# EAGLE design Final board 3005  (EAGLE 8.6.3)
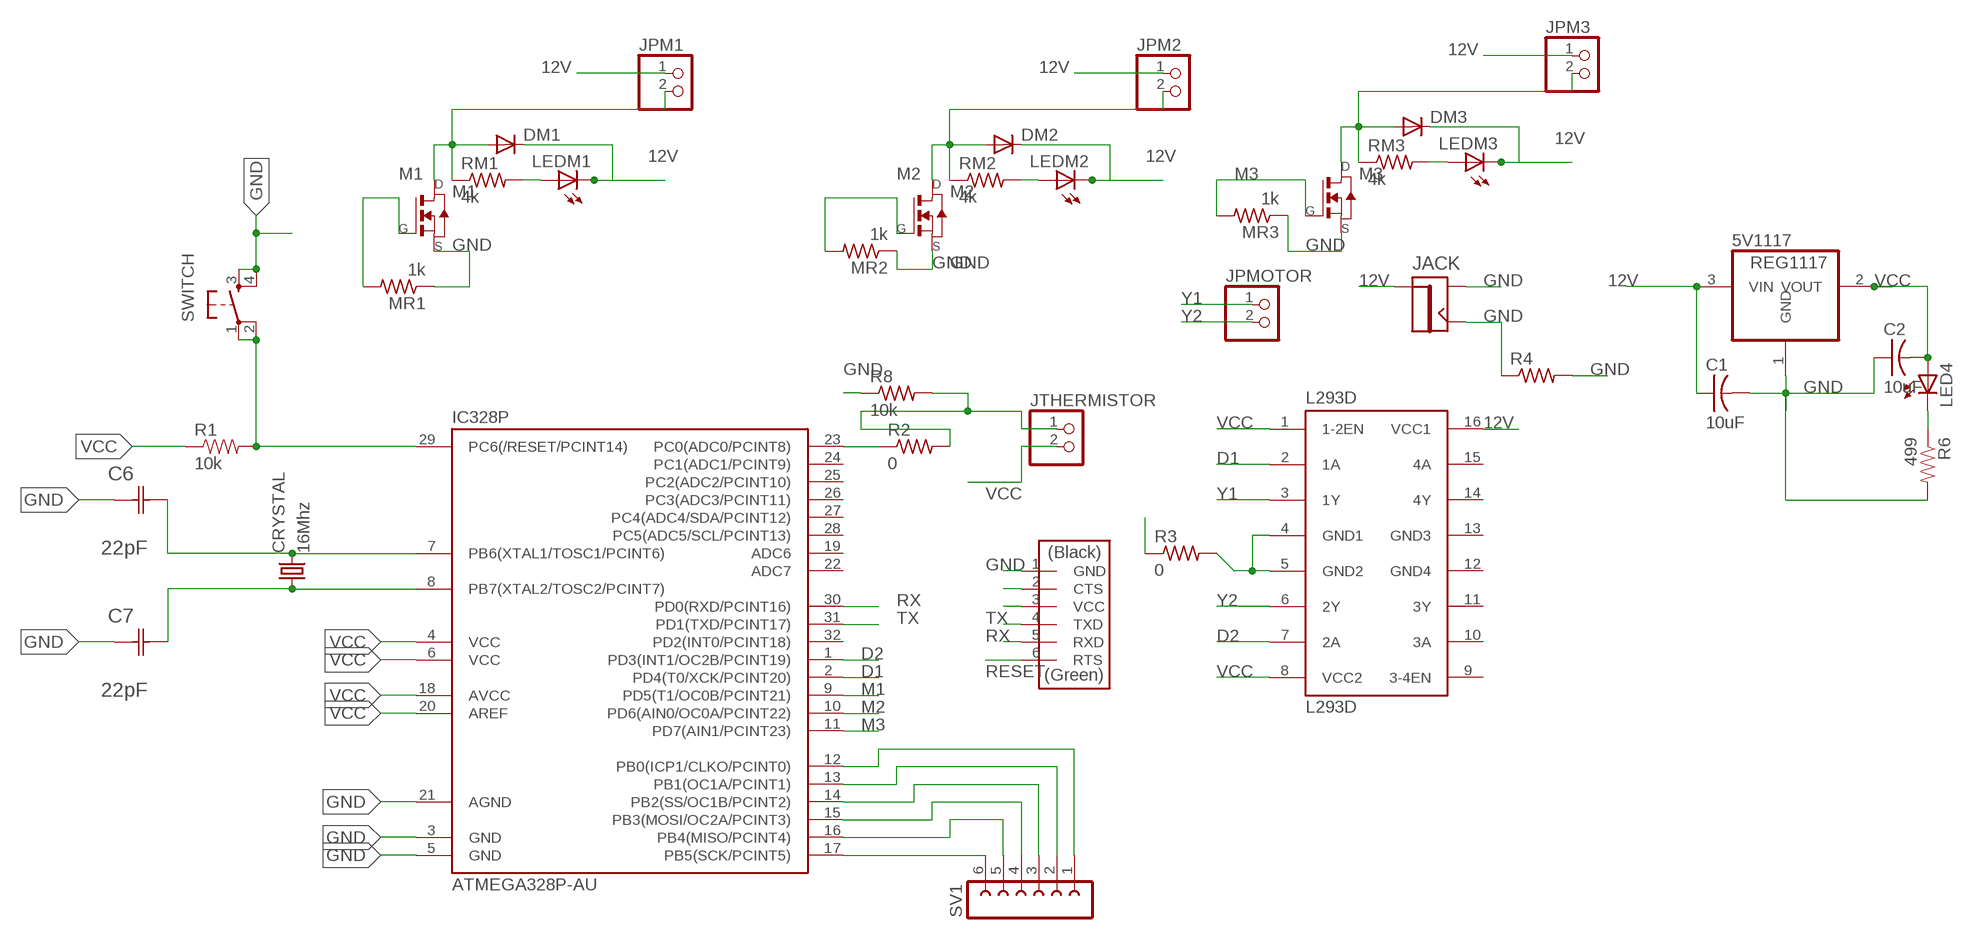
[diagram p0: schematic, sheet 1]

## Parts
5V1117  REG1117  [SOT223]
C1  10uF  CAP-US1206FAB  [C1206FAB]
C2  10uF  CAP-US1206FAB  [C1206FAB]
C6  22pF  0612ZC225MAT2A  [CAPC3216X178N]
C7  22pF  0612ZC225MAT2A  [CAPC3216X178N]
CRYSTAL  16Mhz  CSM-7X-DU  [CSM-7X-DU]
DM1  DIODESOD123  [SOD123]
DM2  DIODESOD123  [SOD123]
DM3  DIODESOD123  [SOD123]
FTDI  FTDI-SMD-HEADER  [1X06SMD]
IC328P  ATMEGA328P-AU  ATMEGA48/88/168-AU  [TQFP32-08]
JACK  JACK2.1MM  [JACK_2.1MM]
JPM1  PINHD-1X2  [1X02]
JPM2  PINHD-1X2  [1X02]
JPM3  PINHD-1X2  [1X02]
JPMOTOR  PINHD-1X2  [1X02]
JTHERMISTOR  PINHD-1X2  [1X02]
L293D  L293D  [DIL16]
LED4  LEDSMT1206  [1206]
LEDM1  LEDSMT1206  [1206]
LEDM2  LEDSMT1206  [1206]
LEDM3  LEDSMT1206  [1206]
M1  NMOSFETTO252  [TO252]
M2  NMOSFETTO252  [TO252]
M3  NMOSFETTO252  [TO252]
MR1  1k  RES-US1206FAB  [R1206FAB]
MR2  1k  RES-US1206FAB  [R1206FAB]
MR3  1k  RES-US1206FAB  [R1206FAB]
R1  10k  RESISTOR1206  [1206]
R2  0  RES-US1206FAB  [R1206FAB]
R3  0  RES-US1206FAB  [R1206FAB]
R4  RES-US1206FAB  [R1206FAB]
R6  499  RESISTOR1206  [1206]
R8  10k  RES-US1206FAB  [R1206FAB]
RM1  4k  RES-US1206  [R1206]
RM2  4k  RES-US1206  [R1206]
RM3  4k  RES-US1206  [R1206]
SV1  FE06-1  [FE06]
SWITCH  6MM_SWITCH6MM_SWITCH  [6MM_SWITCH]

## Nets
12V: 5V1117.3(VIN) C1.1 DM1.CATHODE(C) DM2.CATHODE(C) DM3.CATHODE(C) JACK.PIN JPM1.1 JPM2.1 JPM3.1 L293D.16(VCC1) LEDM1.C LEDM2.C LEDM3.C
D1: IC328P.2(PD4(T0/XCK/PCINT20)) L293D.2(1A)
D2: IC328P.1(PD3(INT1/OC2B/PCINT19)) L293D.7(2A)
GND: 5V1117.1(GND) C1.2 C2.1 C6.1(C1) C7.1(C1) FTDI.1(GND) IC328P.3(GND) IC328P.21(AGND) JACK.CONTACT JACK.SHUNT M1.2(S) M2.2(S) M3.2(S) MR1.1 MR2.1 MR3.1 R3.1 R4.1 R4.2 R6.2 R8.1 SWITCH.3(S) SWITCH.4(S1)
M1: IC328P.9(PD5(T1/OC0B/PCINT21)) M1.1(G) MR1.2
M2: IC328P.10(PD6(AIN0/OC0A/PCINT22)) M2.1(G) MR2.2
M3: IC328P.11(PD7(AIN1/PCINT23)) M3.1(G) MR3.2
MISO: IC328P.16(PB4(MISO/PCINT4)) SV1.5
MOSI: IC328P.15(PB3(MOSI/OC2A/PCINT3)) SV1.4
N$1: LED4.C R6.1
N$2: DM1.ANODE(A) JPM1.2 M1.3(D) RM1.1
N$3: LEDM1.A RM1.2
N$4: C6.2(C2) CRYSTAL.2 IC328P.7(PB6(XTAL1/TOSC1/PCINT6))
N$5: DM2.ANODE(A) JPM2.2 M2.3(D) RM2.1
N$6: LEDM2.A RM2.2
N$7: LEDM3.A RM3.2
N$8: DM3.ANODE(A) JPM3.2 M3.3(D) RM3.1
N$10: IC328P.14(PB2(SS/OC1B/PCINT2)) SV1.3
N$11: C7.2(C2) CRYSTAL.1 IC328P.8(PB7(XTAL2/TOSC2/PCINT7))
N$12: IC328P.12(PB0(ICP1/CLKO/PCINT0)) SV1.1
N$13: IC328P.23(PC0(ADC0/PCINT8)) R2.1
N$14: IC328P.13(PB1(OC1A/PCINT1)) SV1.2
N$16: FTDI.2(CTS)
N$17: L293D.4(GND1) L293D.5(GND2) R3.2
N$30: JTHERMISTOR.1 R2.2 R8.2
RESET: FTDI.6(RTS) IC328P.29(PC6(/RESET/PCINT14)) R1.2 SWITCH.1(P) SWITCH.2(P1)
RX: FTDI.5(RXD) IC328P.30(PD0(RXD/PCINT16))
SCK: IC328P.17(PB5(SCK/PCINT5)) SV1.6
TX: FTDI.4(TXD) IC328P.31(PD1(TXD/PCINT17))
VCC: 5V1117.2(VOUT) C2.2 FTDI.3(VCC) IC328P.6(VCC) IC328P.20(AREF) JTHERMISTOR.2 L293D.1(1-2EN) L293D.8(VCC2) LED4.A R1.1
Y1: JPMOTOR.1 L293D.3(1Y)
Y2: JPMOTOR.2 L293D.6(2Y)
Unconnected: IC328P.18(AVCC) IC328P.19(ADC6) IC328P.22(ADC7) IC328P.24(PC1(ADC1/PCINT9)) IC328P.25(PC2(ADC2/PCINT10)) IC328P.26(PC3(ADC3/PCINT11)) IC328P.27(PC4(ADC4/SDA/PCINT12)) IC328P.28(PC5(ADC5/SCL/PCINT13)) IC328P.32(PD2(INT0/PCINT18)) L293D.9(3-4EN) L293D.10(3A) L293D.11(3Y) L293D.14(4Y) L293D.15(4A)

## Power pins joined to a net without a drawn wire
GND: IC328P.5(GND)
GND3: L293D.13(GND3)
GND4: L293D.12(GND4)
VCC: IC328P.4(VCC)

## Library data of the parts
5V1117 = burr-brown:REG1117: 800mA and 1A Low Dropout (LDO) Positive Regulator 1.8V, 2.5V, 2.85V, 3.3V, 5V, and Adj; MPN: REG1117; OC_FARNELL: 1097566; OC_NEWARK: 14P6981
C1 C2 = fab (1):CAP-US
C6 C7 = AVX_By_element14_Batch_1:0612ZC225MAT2A: Capacitor 1206; MPN: 0612ZC225MAT2A; OC_FARNELL: -; OC_NEWARK: 12N3209; SUPPLIER: AVX; TOLERANCE: ±20%; VALUE: 2.2µF; VOLTAGERATING: 10V
CRYSTAL = 01_FAB_Hello:CSM-7X-DU: SMD CRYSTAL; OC_FARNELL: unknown; OC_NEWARK: unknown
DM1-DM3 = fab (1):DIODE: DIODE
FTDI = fab (1):FTDI-SMD-HEADER
IC328P = atmega8:ATMEGA48/88/168
JACK = fab (1):JACK
JPM1-JPM3 JPMOTOR JTHERMISTOR = pinhead:PINHD-1X2: PIN HEADER
L293D = st-microelectronics:L293D: PUSH-PULL 4 CHANNEL DRIVER; MPN: L293D; OC_FARNELL: 9589619; OC_NEWARK: 56P8249
LED4 LEDM1-LEDM3 = led:LED: LED
M1-M3 = fab (1):NMOSFET: MOS FET
MR1-MR3 R2-R4 R8 RM1-RM3 = fab (1):RES-US: Resistor (US Symbol)
R1 R6 = 01_SparkFun:RESISTOR: Resistor
SV1 = con-lsta:FE06-1: FEMALE HEADER; OC_FARNELL: unknown; OC_NEWARK: unknown
SWITCH = 01_FAB_Hello:6MM_SWITCH: OMRON SWITCH

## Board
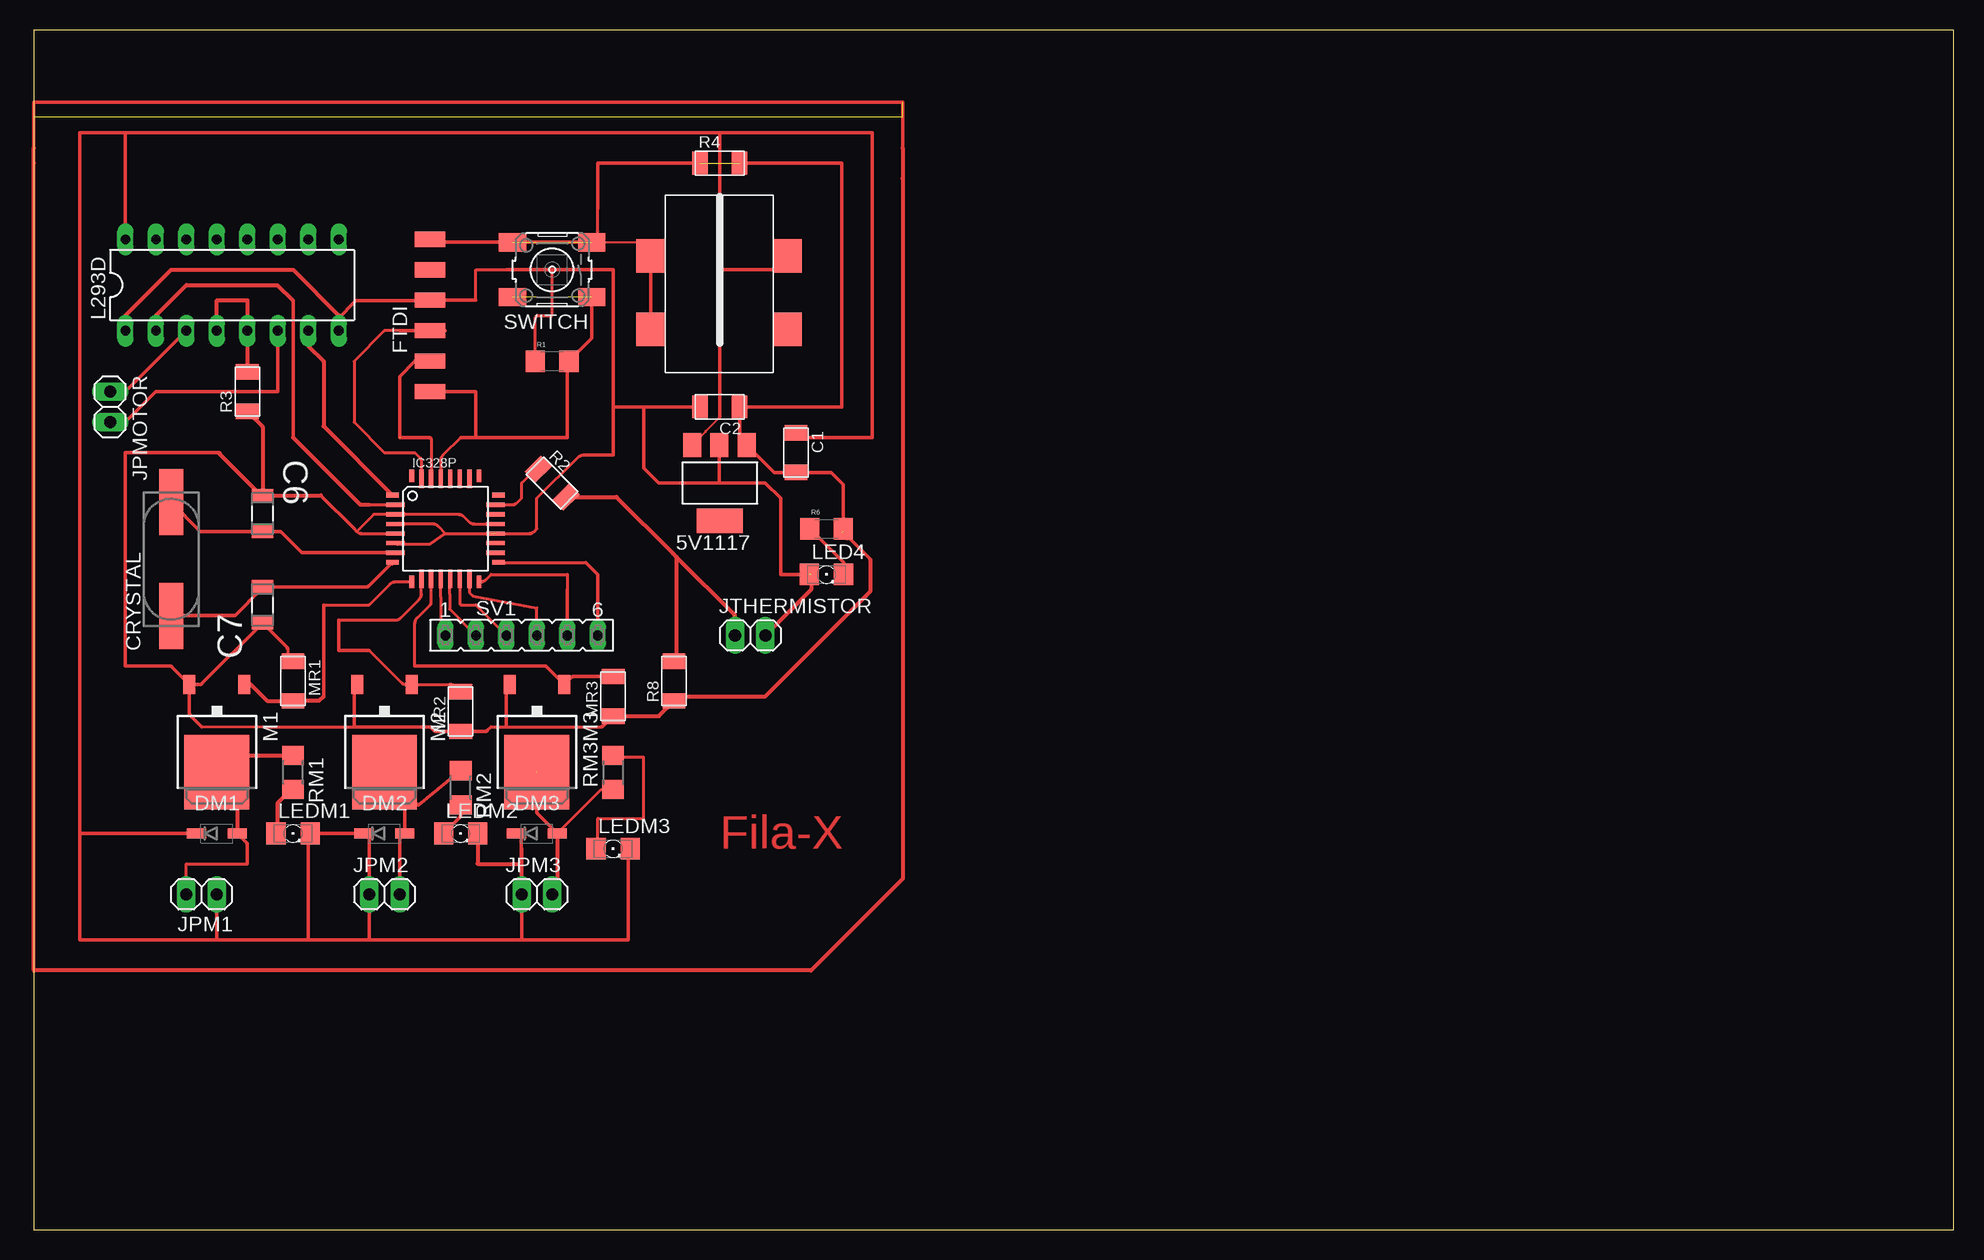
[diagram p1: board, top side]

Size 160 x 100 mm. Coordinates in mm from the lower left corner, seen from the top.
Outline: 0,0 160,0 160,100 0,100 0,0
Copper layers (1*16): Top 0.035mm / dielectric 1.5mm / Bottom 0.035mm
Design rules "default *": minimum track width 12mil, minimum drill 0.35mm, track to track 12mil, track to pad 12mil, pad to pad 12mil, via to via 12mil, smd to smd 12mil, copper to edge 40mil, drill to drill 6mil, minimum pad ring 10mil, minimum via ring 8mil, stop-mask expansion 4mil, vias tented up to drill 0mil, thermal gap 10mil

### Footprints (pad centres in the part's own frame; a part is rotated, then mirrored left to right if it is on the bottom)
SOT223 = smd 1.499 x 2.007: 1 -2.261,-3.15; 2 0.025,-3.15; 3 2.311,-3.15 | smd 3.81 x 2.007: 4 0,3.15
C1206FAB = smd 1.27 x 1.905: 1 -1.651,0; 2 1.651,0
CAPC3216X178N = smd 1.118 x 1.803: 1 -1.499,0; 2 1.499,0
CSM-7X-DU = smd 5.5 x 2: 1 -4.75,0; 2 4.75,0
SOD123 = smd 1.6 x 0.8: ANODE 1.7,0; CATHODE -1.7,0
1X06SMD = smd 2.54 x 1.27: 1 0,6.35; 2 0,3.81; 3 0,1.27; 4 0,-1.27; 5 0,-3.81; 6 0,-6.35
TQFP32-08 = smd 1.016 x 0.406: 1 -4.42,2.8; 8 -4.42,-2.8; 17 4.42,-2.8; 24 4.42,2.8 | smd 1.524 x 0.356: 2 -4.166,2; 3 -4.166,1.2; 4 -4.166,0.4; 5 -4.166,-0.4; 6 -4.166,-1.2; 7 -4.166,-2; 18 4.166,-2; 19 4.166,-1.2; 20 4.166,-0.4; 21 4.166,0.4; 22 4.166,1.2; 23 4.166,2 | smd 0.406 x 1.016: 9 -2.8,-4.42; 16 2.8,-4.42; 25 2.8,4.42; 32 -2.8,4.42 | smd 0.356 x 1.524: 10 -2,-4.166; 11 -1.2,-4.166; 12 -0.4,-4.166; 13 0.4,-4.166; 14 1.2,-4.166; 15 2,-4.166; 26 2,4.166; 27 1.2,4.166; 28 0.4,4.166; 29 -0.4,4.166; 30 -1.2,4.166; 31 -2,4.166
JACK_2.1MM = smd 2.388 x 2.794: CONTACT 5.766,-2.413; PIN -5.639,-2.413; PIN1 -5.639,3.683; SHUNT 5.766,3.683
1X02 = drill 1.016 long: 1 -1.27,0; 2 1.27,0
DIL16 = drill 0.813 long: 1 -8.89,-3.81; 2 -6.35,-3.81; 3 -3.81,-3.81; 4 -1.27,-3.81; 5 1.27,-3.81; 6 3.81,-3.81; 7 6.35,-3.81; 8 8.89,-3.81; 9 8.89,3.81; 10 6.35,3.81; 11 3.81,3.81; 12 1.27,3.81; 13 -1.27,3.81; 14 -3.81,3.81; 15 -6.35,3.81; 16 -8.89,3.81
1206 = smd 1.6 x 1.803: A -1.422,0; C 1.422,0
TO252 = smd 1 x 1.6: 1 -2.28,-4.8; 2 2.28,-4.8 | smd 5.4 x 6.2: 3 0,2.5
R1206FAB = smd 1.27 x 1.905: 1 -1.651,0; 2 1.651,0
1206' = smd 1.6 x 1.8: 1 -1.4,0; 2 1.4,0
R1206 = smd 1.6 x 1.803: 1 -1.422,0; 2 1.422,0
FE06 = drill 0.813 long: 1 -6.35,0; 2 -3.81,0; 3 -1.27,0; 4 1.27,0; 5 3.81,0; 6 6.35,0
6MM_SWITCH = smd 2.286 x 1.524: 1 -3.302,2.286; 2 3.302,2.286; 3 -3.302,-2.286; 4 3.302,-2.286

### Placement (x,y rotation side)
5V1117  57.15,62.23 180 top
C1  63.5,64.77 270 top
C2  57.15,68.58 180 top
C6  19.05,59.69 270 top
C7  19.05,52.07 90 top
CRYSTAL  11.43,55.88 90 top
DM1  15.24,33.02 0 top
DM2  29.21,33.02 0 top
DM3  41.91,33.02 0 top
FTDI  33.02,76.2 0 top
IC328P  34.29,58.42 0 top
JACK  57.15,78.74 180 top
JPM1  13.97,27.94 180 top
JPM2  29.21,27.94 0 top
JPM3  41.91,27.94 0 top
JPMOTOR  6.35,68.58 270 top
JTHERMISTOR  59.69,49.53 0 top
L293D  16.51,78.74 0 top
LED4  66.04,54.61 0 top
LEDM1  21.59,33.02 0 top
LEDM2  35.56,33.02 0 top
LEDM3  48.26,31.75 0 top
M1  15.24,40.64 180 top
M2  29.21,40.64 180 top
M3  41.91,40.64 180 top
MR1  21.59,45.72 270 top
MR2  35.56,43.18 90 top
MR3  48.26,44.45 90 top
R1  10k  [1206']  43.18,72.39 0 top
R2  43.18,62.23 315 top
R3  17.78,69.85 90 top
R4  57.15,88.9 0 top
R6  499  [1206']  66.04,58.42 0 top
R8  53.34,45.72 90 top
RM1  21.59,38.1 270 top
RM2  35.56,36.83 270 top
RM3  48.26,38.1 90 top
SV1  40.64,49.53 0 top
SWITCH  43.18,80.01 180 top

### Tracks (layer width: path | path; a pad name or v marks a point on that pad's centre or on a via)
12V
  Top 0.152: 62.79,80.01 JACK.PIN | 57.15,91.44 57.15,80.01
  Top 0.203: 5V1117.3 55.97,66.51 55.97,66.55 57.15,67.73 57.15,67.77
  Top 0.254: 49.53,31.75 LEDM3.C
  Top 0.305: 22.84,32.95 arc-45 LEDM1.C | LEDM1.C DM2.CATHODE 27.87,32.66 arc-45 27.94,32.48 JPM2.1 27.94,24.13 | 40.62,31.75 40.62,32.51 arc45 40.54,32.69 DM3.CATHODE | C1.1 63.5,66.04 69.85,66.04 69.85,91.44 57.15,91.44 | LEDM3.C 49.53,31.6 49.53,24.13 40.64,24.13 | 40.64,24.13 27.94,24.13 | 27.94,24.13 22.86,24.13 | 22.86,24.13 15.24,24.13 | 15.24,24.13 3.81,24.13 3.81,33.02 | LEDM1.C 22.86,32.87 22.86,24.13 | DM1.CATHODE 3.81,33.02 | JPM1.1 15.24,24.13 | JPM3.1 40.64,24.13 | 7.62,91.44 3.81,91.44 3.81,33.02 | 7.62,91.44 57.15,91.44 | L293D.16 7.62,91.44 | 57.15,91.44 57.15,67.77 | 57.15,80.01 62.79,80.01 | 36.98,30.48 arc-45 36.98,30.48
  Top 0.33: LEDM2.C 36.98,30.48 | 36.98,30.48 | 40.62,31.75 40.62,30.48 | 40.62,30.48 40.62,27.96 JPM3.1 | 36.98,30.48 40.62,30.48
D1
  Top 0.254: 20.27,78.74 20.3,78.72 | 27.94,60.42 IC328P.2
  Top 0.305: L293D.2 10.67,75.44 | 21.59,77.42 21.59,66.04
  Top 0.33: L293D.2 10.16,76.2 12.7,78.74 12.72,78.72 20.3,78.72 21.59,77.42 | 21.59,66.04 27.21,60.42 27.94,60.42
D2
  Top 0.33: L293D.7 22.86,73.66 24.13,72.39 24.13,66.96 IC328P.1
GND  (3 unrouted)
  Top 0.152: SWITCH.3 50.24,82.3 JACK.CONTACT
  Top 0.203: 13.97,41.91 19.05,41.91
  Top 0.254: 19.05,41.91 26.67,41.91 | 47.27,41.91 39.37,41.91 38.1,41.91 37.79,41.6 arc-45 37.61,41.53 | IC328P.21 36.69,58.82 arc-45 36.24,59.01 35.8,59.45 arc45 35.39,59.62 IC328P.3 28.3,59.62 26.88,58.21 | 26.67,58.42 26.88,58.21 | 26.88,58.21 arc45 27.33,58.02 IC328P.5 | 21.14,48.38 21.14,47.83 MR1.1 | SWITCH.3 46.99,82.8 46.99,85.09
  Top 0.305: FTDI.1 33.27,82.3 SWITCH.3 | 23.9,61.19 26.67,58.42 | 67.78,57.62 67.15,58.26 | 5V1117.1 59.56,65.22 arc45 59.74,65.15 | 5V1117.1 58.88,65.92 arc-45 58.8,66.09 C2.1 67.31,68.58 67.31,88.9 R4.2 | 15.54,64.7 arc45 15.36,64.77 7.62,64.77 7.62,46.99 11.3,46.99 arc-45 11.48,46.92 M1.2 | 19.05,50.8 C7.1 | M3.2 39.63,45.72 | 39.63,45.72 39.63,45.88 arc-45 39.7,46.05 | M1.2 13.81,45.44 arc45 13.99,45.51 C7.1 | C7.1 21.06,48.56 arc-45 21.14,48.38 | MR3.1 47.45,41.98 arc-45 47.27,41.91 | 39.37,41.91 39.37,45.35 arc-45 39.44,45.53 39.63,45.72 | 37.79,41.6 arc-45 37.61,41.53 MR2.1 33.51,41.53 arc-45 33.33,41.6 33.02,41.91 26.67,41.91 26.67,45.08 arc-45 26.74,45.25 M2.2 | M1.2 12.96,43.02 arc45 13.03,42.85 13.97,41.91 | 69.69,55.88 67.44,58.13 R6.2 67.44,62.1 66.42,63.12 C1.2 61.67,63.12 5V1117.1 | 46.99,85.09 46.99,88.9 R4.1 | JACK.SHUNT JACK.CONTACT
  Top 0.33: 67.31,58.1 67.78,57.62 | 69.69,55.88 69.69,53.18 60.96,44.45 53.72,44.45 R8.1 52.07,42.8 MR3.1 | R3.1 19.05,66.93 C6.1 | 15.36,64.77 18.95,61.19 C6.1 | C6.1 23.9,61.19
M1
  Top 0.254: 24.13,52.07 27.94,52.07 29.68,53.81 arc-45 30.13,54 IC328P.9
  Top 0.305: 24.13,52.07 24.13,44.45
  Top 0.33: 24.13,44.45 23.75,44.07 MR1.2 19.43,44.07 18.06,45.44 M1.1
M2
  Top 0.254: MR2.2 35.14,45.25 arc45 34.69,45.44 31.75,45.44 M2.1 31.02,45.44 arc-45 30.57,45.63 27.94,48.26 | 25.4,50.8 30.11,50.8 arc45 30.56,50.99 32.1,52.53 arc45 32.29,52.98 IC328P.10
  Top 0.305: 27.94,48.26 25.4,48.26 25.4,50.8
M3
  Top 0.254: IC328P.11 33.09,52.24 arc-45 33.02,52.07 31.94,50.99 arc45 31.75,50.54 31.75,46.99
  Top 0.305: 31.75,46.99 42.53,46.99 arc-45 42.71,46.92 M3.1 44.78,46.03 arc-45 44.96,46.1 MR3.2
MISO
  Top 0.254: IC328P.16 37.23,54 arc45 37.68,54.19 38.1,54.61 44.45,54.61 44.45,53.34
  Top 0.305: 44.45,53.34 SV1.5
MOSI
  Top 0.254: SV1.4 41.91,51.82 36.58,52.83 36.29,53.12 IC328P.15
N$1
  Top 0.305: R6.1 67.46,55.6 LED4.C
N$2
  Top 0.254: JPM1.2 12.7,30.48 17.78,30.48
  Top 0.305: M1.3 16.55,39.45 arc-45 16.73,39.52 | 20.32,39.52 RM1.1 | 13.54,36.3 arc-45 13.61,36.47 15.24,38.1 M1.3 | M1.3 16.87,36.51 arc-45 16.94,36.34 | 17.78,30.48 17.78,32.08 arc45 17.71,32.25 DM1.ANODE
  Top 0.33: RM1.1 16.62,39.52 M1.3 16.94,36.44 DM1.ANODE
N$3
  Top 0.33: LEDM1.A 20.32,33.17 20.32,35.56 21.44,36.68 RM1.2
N$4
  Top 0.305: CRYSTAL.2 13.87,58.19 C6.2 20.55,58.19 22.32,56.42 IC328P.7
N$5
  Top 0.305: M2.3 30.84,36.51 | 30.84,36.51 31.87,35.48 arc45 32.05,35.41 RM2.1 | JPM2.2 30.48,32.48 arc-45 30.55,32.66 DM2.ANODE 30.91,36.34 arc45 30.84,36.51
N$6
  Top 0.305: LEDM2.A 35.49,34.37 arc45 35.56,34.55 RM2.2
N$7
  Top 0.254: LEDM3.A 46.99,31.9 46.99,34.29 50.8,34.29 50.8,39.37 48.41,39.37 RM3.2
N$8  (1 unrouted)
  Top 0.254: DM3.ANODE 47.27,36.68 RM3.1
  Top 0.305: JPM3.2 43.54,28.3 arc45 43.61,28.48 | DM3.ANODE 41.98,34.65 arc-45 41.91,34.83 41.91,38.1
  Top 0.33: DM3.ANODE 43.61,28.37 JPM3.2
N$10
  Top 0.254: IC328P.14 35.49,52.14 35.56,52.07 36.83,52.07 SV1.3
N$11
  Top 0.305: 29.87,55.47 IC328P.8 27.89,53.64 arc-45 27.71,53.57 C7.2 | 19.2,53.65 C7.2 | CRYSTAL.1 11.58,51.21 16.76,51.21 18.9,53.34 C7.2
N$12
  Top 0.254: IC328P.12 33.89,52.73 33.89,49.93 SV1.1
N$13
  Top 0.254: IC328P.23 39.84,60.42 arc45 40.29,60.61 40.64,60.96 40.64,62.23 41.66,63.25 arc-45 R2.1
  Top 0.305: 41.91,63.5 R2.1 41.27,63.4
N$14
  Top 0.254: IC328P.13 arc45 34.64,54.13 34.64,53.34 34.64,52.99 34.64,51.72 SV1.2
N$17
  Top 0.254: 17.78,76.2 L293D.5
  Top 0.305: 15.62,74.55 L293D.4
  Top 0.33: 17.5,74.95 L293D.5 | L293D.4 15.24,77.47 17.78,77.47 L293D.5 | L293D.5 R3.2
N$20  (2 unrouted)
  Top 0.305: 0,90.17 0,92.71 0,93.98 72.39,93.98 72.39,87.63
  Top 0.33: 72.39,90.17 72.39,87.63 72.39,29.21 64.77,21.59 0,21.59 0,88.9 0,90.17
N$30  (1 unrouted)
  Top 0.305: 53.27,56.34 53.34,56.26 | 58.35,51.15 arc-45 58.42,50.97 58.42,48.26
  Top 0.33: JTHERMISTOR.1 58.42,51.18 53.53,56.07 | 53.53,56.07 53.27,56.34 48.54,61.06 R2.2 | 53.53,56.07 53.53,47.56 R8.2
RESET  (1 unrouted)
  Top 0.254: 35.56,66.04 34.08,64.56 arc45 33.89,64.11 IC328P.29
  Top 0.305: SWITCH.1 46.48,74.29 R1.2 44.45,72.26 44.45,66.04 36.83,66.04 | 36.83,66.04 35.56,66.04 | IC328P.29 33.89,63.27 | FTDI.6 36.83,69.85 36.83,66.04
RX  (1 unrouted)
  Top 0.254: 33.02,66.04 arc-45 33.09,65.87 IC328P.30
  Top 0.305: 33.22,72.54 FTDI.5 31.75,72.39 30.48,71.12 30.48,66.04 | 30.54,66.04 33.02,66.04
SCK
  Top 0.254: IC328P.17 45.98,55.62
  Top 0.305: 45.98,55.62 46.99,54.61 SV1.6
TX
  Top 0.254: 30.48,74.93 29.21,74.93 26.67,72.39 26.67,67.31 29.21,64.77 31.75,64.77 32.1,64.42 arc-45 32.29,63.97 IC328P.31
  Top 0.305: 32.92,74.98 FTDI.4 | FTDI.4 30.48,74.93 | 34.29,74.93 FTDI.4
VCC  (2 unrouted)
  Top 0.254: 36.83,77.47 36.83,80.01 40.64,80.01 | 41.91,72.52 R1.1 41.78,76.07 41.91,76.2 43.18,76.2 43.18,80.01 | 34.29,58.02 33.02,57.15 30.29,57.15 arc-45 IC328P.6 | 34.29,58.02 33.68,58.63 arc45 33.23,58.82 IC328P.4 | 34.29,58.02 38.1,58.02 arc-45 38.15,58.04 | IC328P.20 41.25,58.02 arc45 41.7,58.21 41.91,58.42 41.91,60.96 45.32,64.37 arc-45 45.77,64.55 46.99,64.55
  Top 0.305: 25.3,75.89 25.3,74.98 L293D.8 25.3,75.89 | 7.62,74.98 L293D.1 | 25.3,75.89 26.82,77.42 32.92,77.42 FTDI.3 36.83,77.47 | IC328P.4 30.15,58.8 30.48,58.8 | 45.78,64.55 46.99,64.55 48.26,64.55 48.26,68.58 | 39.37,80.01 40.64,80.01 43.18,80.01 48.26,80.01 48.26,68.58 | 41.91,72.39 R1.1 | JTHERMISTOR.2 60.7,50.8 arc45 60.88,50.87 | 5V1117.2 57.12,62.26 57.15,62.23 | 57.15,62.23 60.96,62.23 62.23,60.96 62.23,54.61 64.77,54.61 | 48.26,68.58 50.8,68.58 | 50.8,68.58 C2.2 | 50.8,68.58 50.8,63.5 52.07,62.23 57.15,62.23
  Top 0.33: JTHERMISTOR.2 64.77,53.34 64.77,54.61 | L293D.1 7.62,76.2 11.43,80.01 21.59,80.01 25.4,76.2 L293D.8
Y1
  Top 0.305: JPMOTOR.1 7.62,69.85 L293D.3
Y2
  Top 0.305: 20.12,74.68 L293D.6 20.32,69.85 10.16,69.85 7.62,67.31 JPMOTOR.2

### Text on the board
Top: Fila-X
